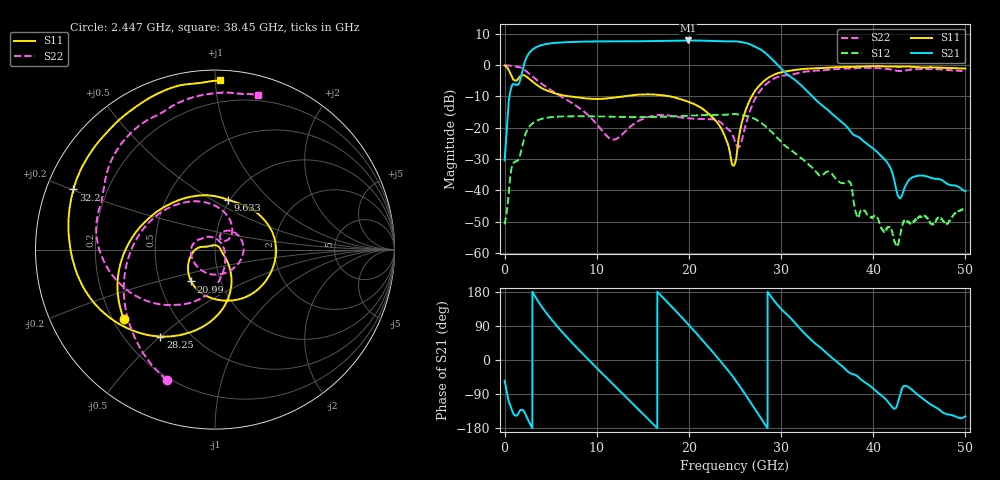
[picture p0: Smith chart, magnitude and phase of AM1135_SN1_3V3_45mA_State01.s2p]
!Agilent Technologies,E8364B,MY43040894,A.07.50.67
!Agilent E8364B: A.07.50.67
!Date: Monday, November 15, 2021 11:26:05
!Correction: S11(Full 2 Port(1,2))
!S21(Full 2 Port(1,2))
!S12(Full 2 Port(1,2))
!S22(Full 2 Port(1,2))
!S2P File: Measurements: S11, S21, S12, S22:
# Hz S  dB  R 50
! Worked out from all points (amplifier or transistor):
!   6401 points, 10 MHz to 50 GHz, reference 50 ohm
!   highest |S21| = 7.8 dB at 19.91 GHz (marker M1)
!   |S21| within 3 dB of that: 2.996 GHz to 27.85 GHz (24.85 GHz wide, 161 % of centre)
!   unconditionally stable (mu >= 1): start of sweep to end of sweep
!   at 8.336 GHz: K = 1.40, MAG = 8.1 dB, |S12| = -16.4 dB
!   at 25 GHz: K = 1.46, MAG = 7.6 dB, |S12| = -15.7 dB
!   at 50 GHz: K = 707.66, MAG = -28.8 dB, |S12| = -45.8 dB
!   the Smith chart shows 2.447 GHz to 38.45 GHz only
!   S11 on the Smith chart (normalised r, x): 2.447 GHz: 0.24, -0.32; 9.633 GHz: 0.98, +0.59; 20.99 GHz: 0.72, -0.27; 28.25 GHz: 0.35, -0.50; 32.2 GHz: 0.08, +0.20; 38.45 GHz: 0.06, +1.03
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1e7  -0.17 -10.6  -30.45 -54.7  -50.91 -52.4  -0.04 -4.6
6.817406e8  -2.97 -59.5  -7.81 -123.5  -34.41 102.4  -0.29 -29.9
2.447012e9  -3.88 -142.5  2.76 -152.7  -20.86 47.7  -2.22 -110.4
3.657708e9  -6.68 170.9  5.97 154.4  -17.57 -7.2  -5.17 -157.1
5.383925e9  -9.00 133.4  7.02 98.3  -16.58 -62.1  -8.72 145.8
8.34427e9  -10.52 90.1  7.43 19.8  -16.37 -135.6  -14.20 67.3
9.633075e9  -10.83 75.4  7.50 -12.1  -16.40 -164.9  -17.65 44.0
1.149208e10  -10.55 55.7  7.56 -57.3  -16.51 154.1  -23.57 47.9
1.306208e10  -10.00 35.5  7.56 -95.1  -16.60 120.3  -21.33 70.6
1.667854e10  -9.53 -29.1  7.66 177.5  -16.58 43.1  -16.01 13.6
1.991227e10  -11.69 -102.3  7.83 94.7  -16.20 -30.2  -17.01 -80.4
2.099018e10  -13.08 -127.0  7.81 65.6  -16.08 -56.2  -17.23 -117.7
2.309913e10  -18.46 -175.4  7.67 6.5  -15.91 -109.8  -17.71 172.0
2.5005e10  -31.47 30.7  7.55 -51.5  -15.66 -164.6  -24.34 82.9
2.639535e10  -12.61 -67.9  6.85 -100.8  -16.38 148.7  -16.71 -74.4
2.825435e10  -4.86 -122.1  3.92 -169.8  -19.43 83.0  -6.50 -142.6
2.966813e10  -2.59 -157.8  -0.09 143.9  -23.45 40.5  -3.80 179.7
3.219887e10  -1.34 157.0  -6.55 79.2  -29.77 -12.5  -2.35 138.8
3.333927e10  -1.11 141.5  -9.84 51.4  -32.69 -35.2  -1.88 123.8
3.844762e10  -0.51 88.3  -23.08 -46.4  -48.39 -114.0  -0.95 74.6
4.167354e10  -0.51 57.1  -31.81 -112.6  -51.75 -122.8  -1.32 43.5
5e10  -1.13 -61.3  -40.34 -148.6  -45.83 -106.5  -1.57 -70.7
